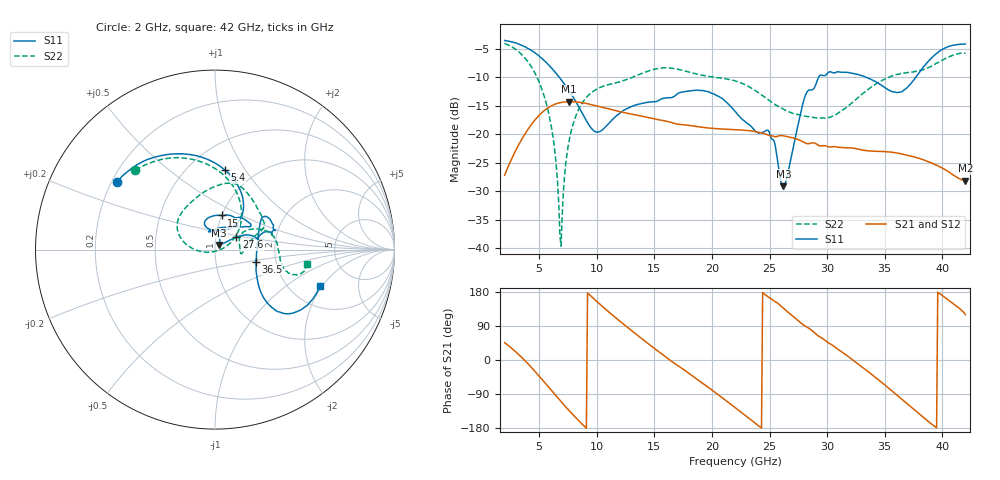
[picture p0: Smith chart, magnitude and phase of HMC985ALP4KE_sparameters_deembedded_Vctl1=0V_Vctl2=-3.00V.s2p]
!s2p File: Measurements: S11, S21, S12, S22
# GHz S dB R 50.0
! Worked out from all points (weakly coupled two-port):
!   401 points, 2 GHz to 42 GHz, reference 50 ohm
!   highest |S21| = -14.27 dB at 7.6 GHz (marker M1); lowest = -28.1 dB at 42 GHz (marker M2)
!   lowest |S11| = -29.1 dB at 26.2 GHz (marker M3), VSWR 1.07, Z = 52.3 + j2.78 ohm
!   |S11| at or under -10 dB: 6.752 GHz to 29.26 GHz (22.5 GHz wide, 125 % of centre); 33.39 GHz to 37.7 GHz (4.302 GHz wide, 12.1 % of centre)
!   |S22| runs from -39.6 to -4.1 dB; largest |S21 - S12| = 0.00068
!   S11 on the Smith chart (normalised r, x): 2 GHz: 0.22, +0.30; 5.4 GHz: 0.73, +0.81; 15 GHz: 1.00, +0.39; 27.6 GHz: 1.26, +0.18; 36.5 GHz: 1.57, -0.22; 42 GHz: 2.92, -1.90
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2  -3.54 145.4  -27.18 45.6  -27.16 45.7  -4.07 135.1
3.5  -4.40 119.4  -20.83 6.4  -20.85 6.4  -6.05 99.7
5.4  -6.99 83.0  -15.90 -56.8  -15.93 -56.8  -13.08 48.6
6.2  -8.65 68.7  -14.86 -85.4  -14.84 -85.4  -20.42 24.0
6.8  -10.12 59.6  -14.45 -106.5  -14.46 -106.6  -37.57 -30.8
7  -10.65 57.1  -14.37 -113.4  -14.39 -113.5  -34.19 -139.2
7.6  -12.36 51.8  -14.27 -133.6  -14.28 -133.6  -21.11 -174.5
8.7  -16.15 53.3  -14.43 -168.1  -14.44 -168.1  -14.62 164.8
10.1  -19.60 87.7  -15.06 151.7  -15.04 151.8  -11.96 146.8
15  -14.26 79.2  -17.28 30.4  -17.27 30.4  -8.59 81.6
15.4  -14.03 74.4  -17.47 21.5  -17.50 21.5  -8.43 77.9
19.3  -12.35 33.7  -18.79 -63.7  -18.80 -63.7  -9.68 42.2
22  -15.94 52.0  -19.17 -125.3  -19.19 -125.3  -10.63 23.8
25  -19.75 99.6  -20.23 164.1  -20.20 164.1  -14.10 11.9
26.2  -29.11 49.3  -20.25 136.7  -20.28 136.6  -15.60 -0.2
27.6  -17.20 30.0  -21.00 100.5  -21.04 100.5  -16.55 -8.8
28.7  -12.20 13.0  -21.50 77.3  -21.48 77.3  -16.99 -4.5
31  -9.06 23.2  -22.26 27.1  -22.24 27.0  -16.20 26.8
35.4  -12.26 11.8  -23.07 -75.8  -23.07 -75.9  -9.96 16.9
36.5  -12.51 -16.5  -23.44 -104.2  -23.45 -104.3  -9.29 9.1
39.5  -5.84 -43.5  -25.39 -178.9  -25.39 -178.9  -7.53 -16.9
42  -4.16 -18.9  -28.11 119.6  -28.12 119.6  -5.72 -8.9
